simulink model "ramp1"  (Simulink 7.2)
settings: Solver=ode45  StartTime=0.0  StopTime=10.0  RelTol=1e-3
undefined symbols (not defined in the file or in its folder): a
libraries: simulink x1

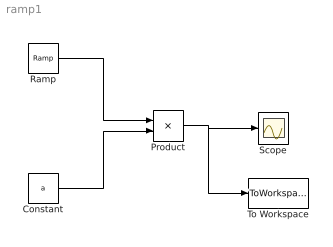
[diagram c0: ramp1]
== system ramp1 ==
  Constant : Constant  Value=a  OutDataType=sfix(16)  OutScaling=2^0
  Product : Product  OutDataType=sfix(16)  OutScaling=2^0
  Ramp : simulink/Sources/Ramp  SystemSampleTime=-1  slope=1  start=0  X0=0
  Scope : Scope
  To Workspace : ToWorkspace  VariableName=var  SampleTime=-1  SaveFormat=Structure
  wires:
  Ramp/1 -> Product/1
  Product/1 -> Scope/1, To Workspace/1
  Constant/1 -> Product/2
